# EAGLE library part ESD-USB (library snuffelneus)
4 DIODES SIL, common cathode
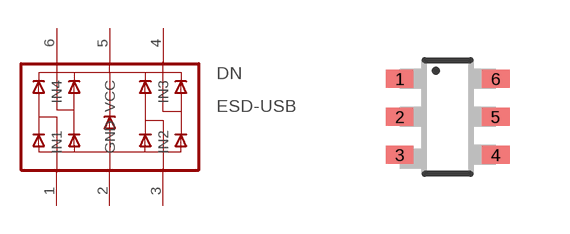
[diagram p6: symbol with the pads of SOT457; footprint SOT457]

Designator prefix DN

## ESD-USBSOT457  [SOT457]
1  IN1
2  GND
3  IN2
4  IN3
5  VCC
6  IN4

## Footprint SOT457 (pad centres in mm)
Small Outline Transistor 6 lead
smd 0.7 x 0.45: 1 -1.2,0.95; 2 -1.2,0; 3 -1.2,-0.95; 4 1.2,-0.95; 5 1.2,0; 6 1.2,0.95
